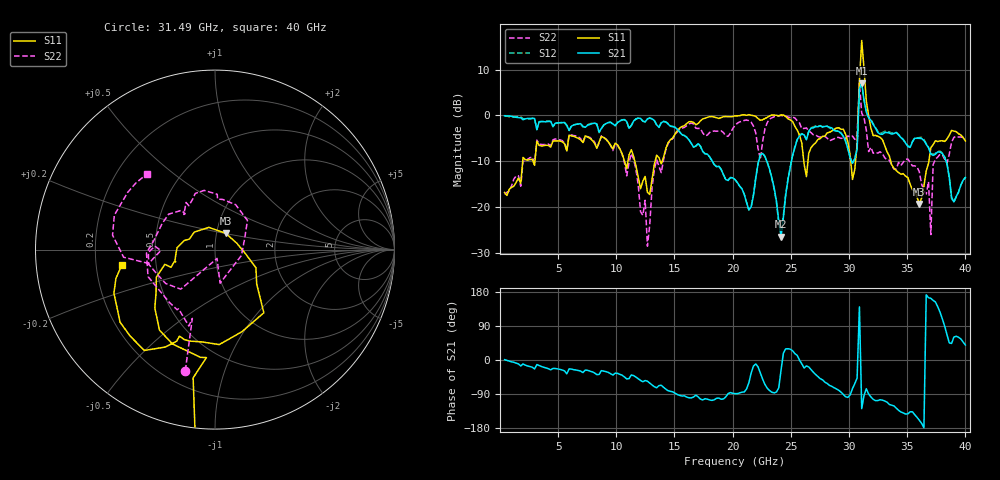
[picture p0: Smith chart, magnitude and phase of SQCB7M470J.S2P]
! Network Analyzer HP8722ES.07.66: Jul 25, 2000 Serial No. US39175408
! 27 Oct 2004  10:50:52
! Frequency  S11  S21  S12  S22
# HZ  S  DB R  50
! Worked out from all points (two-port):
!   201 points, 400 MHz to 40 GHz, reference 50 ohm
!   highest |S21| = 7.03 dB at 31.09 GHz (marker M1); lowest = -26.4 dB at 24.16 GHz (marker M2)
!   |S21| within 3 dB of the highest: 30.87 GHz to 31.25 GHz (383.6 MHz wide, 1.24 % of centre)
!   lowest |S11| = -19.3 dB at 36.04 GHz (marker M3), VSWR 1.24, Z = 55.4 + j10.1 ohm
!   |S11| at or under -10 dB: start of sweep to 1.954 GHz; 11.59 GHz to 13.33 GHz (1.741 GHz wide, 14 % of centre); 33.59 GHz to 36.86 GHz (3.268 GHz wide, 9.28 % of centre)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
!   |S22| runs from -28.5 to 7.0 dB; largest |S21 - S12| = 0.17
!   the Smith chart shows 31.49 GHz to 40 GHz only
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4e8  -16.79 -93.6  -0.09 0.9  -0.03 1.9  -17.19 -89.6
7.132e9  -5.92 -106.0  -2.38 -33.1  -2.53 -34.2  -6.03 -118.5
1.129e10  -7.47 -95.6  -2.19 -39.4  -2.19 -39.9  -8.32 -119.7
1.2676e10  -16.73 -62.8  -0.77 -56.0  -0.72 -56.9  -28.48 -111.1
1.3666e10  -9.21 -24.8  -2.61 -67.5  -2.53 -67.3  -11.12 -27.3
2.02e10  -0.10 -8.5  -13.96 -88.8  -13.98 -89.5  -2.18 -17.6
2.2576e10  -0.94 -16.8  -8.28 -50.7  -8.17 -52.4  -5.68 10.9
2.416e10  0.11 -41.9  -26.40 -26.0  -26.34 -21.6  -0.00 -17.7
2.5744e10  -4.28 -131.6  -4.49 -0.3  -4.22 -0.6  -1.64 -35.7
2.6932e10  -6.40 140.5  -2.69 -32.2  -2.50 -33.9  -4.22 -38.9
2.9506e10  -2.99 28.4  -4.47 -91.0  -4.64 -91.1  -4.94 -43.3
3.0694e10  -6.34 74.6  -7.38 -47.7  -7.13 -48.5  -4.29 -102.4
3.0892e10  7.47 -30.5  5.77 140.3  6.49 139.4  7.02 -8.1
3.109e10  16.34 -72.5  7.03 -128.4  6.92 -128.4  0.51 172.3
3.1288e10  10.21 -74.8  3.31 -93.6  3.36 -93.2  -0.49 -128.4
3.1486e10  3.14 -69.6  0.74 -75.9  0.89 -77.0  -3.17 -103.8
3.1684e10  -0.05 -96.5  -0.47 -89.6  -0.46 -90.5  -7.88 -108.2
3.3466e10  -8.85 -154.9  -3.85 -117.4  -3.58 -118.8  -9.75 142.7
3.604e10  -19.28 56.3  -4.99 -158.9  -4.83 -159.0  -12.28 42.0
3.703e10  -7.03 -52.3  -8.43 162.8  -8.25 162.8  -25.95 -76.9
3.7228e10  -6.35 -71.8  -8.71 157.2  -8.48 157.7  -10.71 -130.9
4e10  -5.56 -170.4  -13.51 39.4  -13.49 39.3  -4.93 131.8
